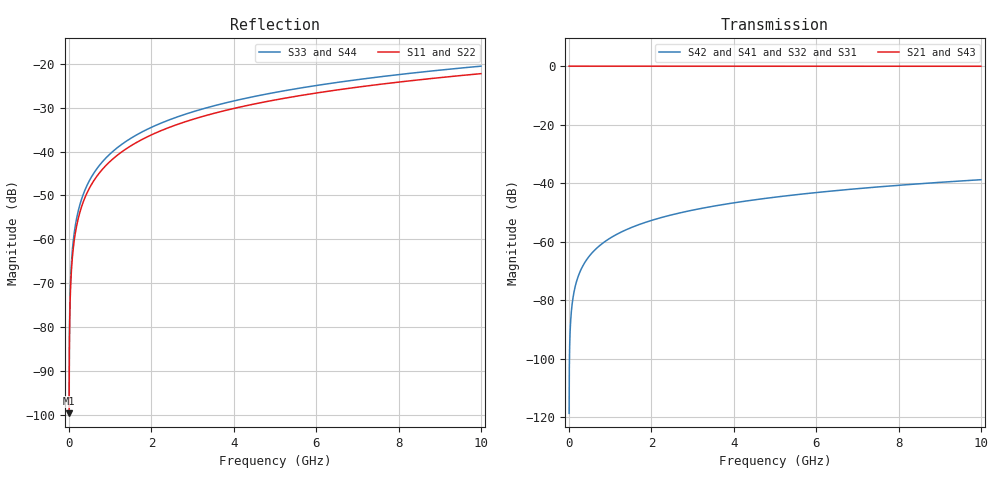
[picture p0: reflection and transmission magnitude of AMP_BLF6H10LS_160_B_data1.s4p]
! Created Thu Oct 06 14:21:55 2011
# ghz S ma R 50
! 4 Port Network Data from SP1.SP block
! freq  magS11  angS11  magS12  angS12  magS13  angS13  magS14  angS14
!  magS21  angS21  magS22  angS22  magS23  angS23  magS24  angS24
!  magS31  angS31  magS32  angS32  magS33  angS33  magS34  angS34
!  magS41  angS41  magS42  angS42  magS43  angS43  magS44  angS44
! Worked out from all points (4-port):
!   10000 points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, 1 MHz to 10 GHz, reference 50 ohm
!   strongest paths, dB at 1 MHz, 2.501 GHz, 5.001 GHz, 7.501 GHz, 10 GHz:
!     S21: 0.0, 0.0, 0.0, 0.0, 0.0
!     S43: 0.0, 0.0, 0.0, 0.0, 0.0
!     S42: -118.6, -50.8, -44.8, -41.3, -38.8
!     S41: -118.6, -50.8, -44.8, -41.3, -38.8
!     S32: -118.6, -50.8, -44.8, -41.3, -38.8
!     S31: -118.6, -50.8, -44.8, -41.3, -38.8
!   lowest |S11| = -99.7 dB at 1 MHz (marker M1), VSWR 1.00, Z = 50 + j0.000786 ohm
!   |S11| at or under -10 dB: start of sweep to end of sweep
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0.001  1.039e-05 49.1  1 -0.0  1.172e-06 -90.4  1.172e-06 89.6
       1 -0.0  1.039e-05 49.1  1.172e-06 89.6  1.172e-06 -90.4
       1.172e-06 -90.4  1.172e-06 89.6  1.619e-05 36.0  1 -0.0
       1.172e-06 89.6  1.172e-06 -90.4  1 -0.0  1.619e-05 36.0
0.118  0.0009148 89.1  1 -0.1  0.0001366 -90.1  0.0001366 89.9
       1 -0.1  0.0009148 89.1  0.0001366 89.9  0.0001366 -90.1
       0.0001366 -90.1  0.0001366 89.9  0.001115 88.7  1 -0.1
       0.0001366 89.9  0.0001366 -90.1  1 -0.1  0.001115 88.7
0.341  0.002643 89.4  1 -0.2  0.0003947 -90.4  0.0003947 89.6
       1 -0.2  0.002643 89.4  0.0003947 89.6  0.0003947 -90.4
       0.0003947 -90.4  0.0003947 89.6  0.003222 89.1  1 -0.2
       0.0003947 89.6  0.0003947 -90.4  1 -0.2  0.003222 89.1
0.798  0.006185 89.3  0.9999 -0.4  0.0009237 -90.8  0.0009237 89.2
       0.9999 -0.4  0.006185 89.3  0.0009237 89.2  0.0009237 -90.8
       0.0009237 -90.8  0.0009237 89.2  0.007539 89.1  0.9999 -0.4
       0.0009237 89.2  0.0009237 -90.8  0.9999 -0.4  0.007539 89.1
1.552  0.01203 89.1  0.9999 -0.7  0.001796 -91.5  0.001796 88.5
       0.9999 -0.7  0.01203 89.1  0.001796 88.5  0.001796 -91.5
       0.001796 -91.5  0.001796 88.5  0.01466 88.8  0.9998 -0.8
       0.001796 88.5  0.001796 -91.5  0.9998 -0.8  0.01466 88.8
4.541  0.03517 87.8  0.9993 -2.0  0.005248 -94.5  0.005248 85.5
       0.9993 -2.0  0.03517 87.8  0.005248 85.5  0.005248 -94.5
       0.005248 -94.5  0.005248 85.5  0.04285 87.3  0.9989 -2.5
       0.005248 85.5  0.005248 -94.5  0.9989 -2.5  0.04285 87.3
10  0.07725 85.4  0.9968 -4.4  0.01149 -99.8  0.01149 80.2
    0.9968 -4.4  0.07725 85.4  0.01149 80.2  0.01149 -99.8
    0.01149 -99.8  0.01149 80.2  0.09401 84.4  0.9952 -5.4
    0.01149 80.2  0.01149 -99.8  0.9952 -5.4  0.09401 84.4
